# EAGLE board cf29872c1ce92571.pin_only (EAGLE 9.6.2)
REV: E

Size 48.26 x 40.64 mm. Coordinates in mm from the lower left corner, seen from the top.
Outline: 2.54,40.64 45.72,40.64 arc-90 48.26,38.1 48.26,2.54 arc-90 45.72,0 2.54,0 arc-90 0,2.54 0,38.1 arc-90 2.54,40.64
Copper layers (1*16): Top 0.035mm / dielectric 1.5mm / Bottom 0.035mm
Design rules "adafruit 8-8": minimum track width 6mil, minimum drill 15.5mil, track to track 8mil, track to pad 8mil, pad to pad 8mil, via to via 8mil, smd to smd 8mil, copper to edge 10mil, drill to drill 8mil, minimum pad ring 10mil, minimum via ring 8mil, stop-mask expansion 2mil, vias tented up to drill 20mil, thermal gap 10mil

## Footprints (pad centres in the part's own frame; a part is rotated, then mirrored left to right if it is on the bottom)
0603-NO = smd 1.075 x 1: 1 -0.85,0; 2 0.85,0
0805-NO = smd 1.24 x 1.5: 1 -0.95,0; 2 0.95,0
SOD-123 = smd 1.4 x 1.4: A 1.85,0; C -1.85,0
SOD-323_MINI = smd 0.9 x 0.8: A 1.07,0; C -1.07,0
FIDUCIAL_1MM = smd 1 x 1: 1 0,0
SOT23-5 = smd 0.69 x 0.99: 1 -0.95,-1.29; 2 0,-1.29; 3 0.95,-1.29; 4 0.95,1.3; 5 -0.95,1.3
FPC_40 = smd 0.275 x 1.2: 1 -9.75,-1.044; 2 -9.25,-1.044; 3 -8.75,-1.044; 4 -8.25,-1.044; 5 -7.75,-1.044; 6 -7.25,-1.044; 7 -6.75,-1.044; 8 -6.25,-1.044; 9 -5.75,-1.044; 10 -5.25,-1.044; 11 -4.75,-1.044; 12 -4.25,-1.044; 13 -3.75,-1.044; 14 -3.25,-1.044; 15 -2.75,-1.044; 16 -2.25,-1.044; 17 -1.75,-1.044; 18 -1.25,-1.044; 19 -0.75,-1.044; 20 -0.25,-1.044; 21 0.25,-1.044; 22 0.75,-1.044; 23 1.25,-1.044; 24 1.75,-1.044; 25 2.25,-1.044; 26 2.75,-1.044; 27 3.25,-1.044; 28 3.75,-1.044; 29 4.25,-1.044; 30 4.75,-1.044; 31 5.25,-1.044; 32 5.75,-1.044; 33 6.25,-1.044; 34 6.75,-1.044; 35 7.25,-1.044; 36 7.75,-1.044; 37 8.25,-1.044; 38 8.75,-1.044; 39 9.25,-1.044; 40 9.75,-1.044 | smd 2.4 x 3.81: PAD1 11.85,1.163; PAD2 -11.85,1.163
1X15-CB = drill 1.016 pad 1.778: 1 -17.78,0; 2 -15.24,0; 3 -12.7,0; 4 -10.16,0; 5 -7.62,0; 6 -5.08,0; 7 -2.54,0; 8 0,0; 9 2.54,0; 10 5.08,0; 11 7.62,0; 12 10.16,0; 13 12.7,0; 14 15.24,0; 15 17.78,0
INDUCTOR_5X5MM_NR5040_NOTHERMALS = smd 1.8 x 4: P$1 -1.8,0; P$2 1.8,0
RESPACK_4X0603 = smd 0.45 x 0.9: 1 -1.3,-0.85; 2 -0.4,-0.85; 3 0.4,-0.85; 4 1.3,-0.85; 5 1.3,0.85; 6 0.4,0.85; 7 -0.4,0.85; 8 -1.3,0.85
SOLDERJUMPER_ARROW_NOPASTE = smd 0.762 x 1.524: 1 -1.016,0; 2 1.016,0
LQFP100 = smd 0.27 x 1.5: 1 -6,-7.75; 2 -5.5,-7.75; 3 -5,-7.75; 4 -4.5,-7.75; 5 -4,-7.75; 6 -3.5,-7.75; 7 -3,-7.75; 8 -2.5,-7.75; 9 -2,-7.75; 10 -1.5,-7.75; 11 -1,-7.75; 12 -0.5,-7.75; 13 0,-7.75; 14 0.5,-7.75; 15 1,-7.75; 16 1.5,-7.75; 17 2,-7.75; 18 2.5,-7.75; 19 3,-7.75; 20 3.5,-7.75; 21 4,-7.75; 22 4.5,-7.75; 23 5,-7.75; 24 5.5,-7.75; 25 6,-7.75; 51 6,7.75; 52 5.5,7.75; 53 5,7.75; 54 4.5,7.75; 55 4,7.75; 56 3.5,7.75; 57 3,7.75; 58 2.5,7.75; 59 2,7.75; 60 1.5,7.75; 61 1,7.75; 62 0.5,7.75; 63 0,7.75; 64 -0.5,7.75; 65 -1,7.75; 66 -1.5,7.75; 67 -2,7.75; 68 -2.5,7.75; 69 -3,7.75; 70 -3.5,7.75; 71 -4,7.75; 72 -4.5,7.75; 73 -5,7.75; 74 -5.5,7.75; 75 -6,7.75 | smd 1.5 x 0.27: 26 7.75,-6; 27 7.75,-5.5; 28 7.75,-5; 29 7.75,-4.5; 30 7.75,-4; 31 7.75,-3.5; 32 7.75,-3; 33 7.75,-2.5; 34 7.75,-2; 35 7.75,-1.5; 36 7.75,-1; 37 7.75,-0.5; 38 7.75,0; 39 7.75,0.5; 40 7.75,1; 41 7.75,1.5; 42 7.75,2; 43 7.75,2.5; 44 7.75,3; 45 7.75,3.5; 46 7.75,4; 47 7.75,4.5; 48 7.75,5; 49 7.75,5.5; 50 7.75,6; 76 -7.75,6; 77 -7.75,5.5; 78 -7.75,5; 79 -7.75,4.5; 80 -7.75,4; 81 -7.75,3.5; 82 -7.75,3; 83 -7.75,2.5; 84 -7.75,2; 85 -7.75,1.5; 86 -7.75,1; 87 -7.75,0.5; 88 -7.75,0; 89 -7.75,-0.5; 90 -7.75,-1; 91 -7.75,-1.5; 92 -7.75,-2; 93 -7.75,-2.5; 94 -7.75,-3; 95 -7.75,-3.5; 96 -7.75,-4; 97 -7.75,-4.5; 98 -7.75,-5; 99 -7.75,-5.5; 100 -7.75,-6
SC70-5 = smd 0.35 x 1.15: 1 -0.65,-0.85; 2 0,-0.85; 3 0.65,-0.85; 4 0.65,0.85; 5 -0.65,0.85
SOT23-5' = smd 0.55 x 1.2: 1 -0.95,-1.3; 2 0,-1.3; 3 0.95,-1.3; 4 0.95,1.3; 5 -0.95,1.3
TSSOP16 = smd 0.305 x 0.991: 1 -2.275,-2.918; 2 -1.625,-2.918; 3 -0.975,-2.918; 4 -0.325,-2.918; 5 0.325,-2.918; 6 0.975,-2.918; 7 1.625,-2.918; 8 2.275,-2.918; 9 2.275,2.918; 10 1.625,2.918; 11 0.975,2.918; 12 0.325,2.918; 13 -0.325,2.918; 14 -0.975,2.918; 15 -1.625,2.918; 16 -2.275,2.918
MOUNTINGHOLE_2.5_PLATED = drill 2.5 pad 3.2: P$1 0,0
CRYSTAL_3.2X2.5 = smd 1.4 x 1.2: 1 -1.1,-0.8; 2 1.1,0.8; GND1 -1.1,0.8; GND2 1.1,-0.8

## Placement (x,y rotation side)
C1  0.1uF  [0603-NO]  15.24,28.07 90 top
C2  15pF  [0603-NO]  9.9,14.73 0 top
C3  15pF  [0603-NO]  13.58,10.67 180 top
C4  1uF  [0805-NO]  13.96,20.95 180 top
C5  0.1uF  [0603-NO]  36.95,17.4 0 top
C6  0.1uF  [0603-NO]  34.92,9.65 0 top
C7  0.1uF  [0603-NO]  16.25,8.38 180 top
C8  0.1uF  [0603-NO]  37.33,23.24 270 top
C9  0.1uF  [0603-NO]  12.44,8.38 180 top
C10  0.1uF  [0603-NO]  13.96,18.8 180 top
C11  0.1uF  [0603-NO]  13.96,17.27 180 top
C12  0.1uF  [0603-NO]  36.82,15.11 0 top
C16  10uF  [0805-NO]  7.87,17.78 0 top
C17  1uF  [0805-NO]  13.6,24.64 270 top
C18  0.1uF  [0603-NO]  2.41,26.3 0 top
C19  10uF  [0805-NO]  2.28,11.43 90 top
C20  1uF  [0805-NO]  16.76,29.72 270 top
C21  10uF  [0805-NO]  14.16,33.07 180 top
C22  10uF  [0805-NO]  8.63,10.67 90 top
D2  MBR0540  [SOD-123]  11.68,24.51 270 top
D3  1N4148  [SOD-323_MINI]  3.3,17.53 90 top
D4  1N4148  [SOD-323_MINI]  1.52,17.53 90 top
FB2  Ferrite  [0805-NO]  6.35,7.87 270 top
FID1  FIDUCIAL_1MM  [FIDUCIAL_1MM]  2.41,7.11 0 top
FID2  FIDUCIAL_1MM  [FIDUCIAL_1MM]  45.97,7.11 0 top
FID3  FIDUCIAL_1MM  [FIDUCIAL_1MM]  46.35,27.56 0 top
IC2  74AHC1G125DBV  [SOT23-5]  41.02,14.61 270 top
J1  40PINFPC_GENERIC  [FPC_40]  28.44,36.07 0 top
JP1  Breakout  [1X15-CB]  24.13,1.91 180 top
L1  6.8uH large inductor  [INDUCTOR_5X5MM_NR5040_NOTHERMALS]  7.36,21.84 90 top
PLABEL0  [PLABEL0]  6.34,3.05 90 top
PLABEL1  [PLABEL1]  8.88,3.05 90 top
PLABEL2  [PLABEL2]  11.42,2.92 90 top
PLABEL3  [PLABEL3]  16.5,2.92 90 top
PLABEL4  [PLABEL4]  19.04,2.92 90 top
PLABEL5  [PLABEL5]  21.58,3.05 90 top
PLABEL6  [PLABEL6]  24.12,3.05 90 top
PLABEL7  [PLABEL7]  26.66,3.05 90 top
PLABEL8  [PLABEL8]  29.2,3.05 90 top
PLABEL9  [PLABEL9]  31.74,3.05 90 top
PLABEL10  [PLABEL10]  5.46,37.47 0 top
PLABEL11  [PLABEL11]  1.27,34.54 0 top
PLABEL12  [PLABEL12]  1.65,30.99 0 top
PLABEL13  [PLABEL13]  34.28,3.05 90 top
PLABEL14  [PLABEL14]  36.82,3.05 90 top
PLABEL15  [PLABEL15]  39.36,3.05 90 top
PLABEL16  [PLABEL16]  41.9,3.05 90 top
PLABEL17  [PLABEL17]  13.96,3.05 90 top
PLABEL18  [PLABEL18]  5.33,26.42 0 top
PLABEL19  [PLABEL19]  2.29,32.89 0 top
PLABEL20  [PLABEL20]  9.02,26.42 0 top
PLABEL21  [PLABEL21]  30.1,34.67 0 bottom
PLABEL22  [PLABEL22]  24.77,24.13 0 bottom
PLABEL23  [PLABEL23]  25.02,13.34 0 bottom
R1  2Ω  [0805-NO]  10.67,29.08 90 top
R3  1M  [0603-NO]  10.66,11.68 90 top
R4  33  [RESPACK_4X0603]  32.5,29.21 0 top
R5  33  [RESPACK_4X0603]  28.44,29.21 0 top
R6  33  [RESPACK_4X0603]  24.38,29.21 0 top
R7  33  [RESPACK_4X0603]  20.31,29.46 0 top
R8  33  [RESPACK_4X0603]  36.57,29.21 0 top
R9  8.2Ω  [0805-NO]  6.73,28.96 90 top
R10  8.2Ω  [0805-NO]  2.67,28.96 90 top
R11  10K  [0603-NO]  2.4,20.57 0 top
R12  10K  [0603-NO]  38.98,10.41 90 top
SJ1  +25mA  [SOLDERJUMPER_ARROW_NOPASTE]  4.7,28.96 90 top
SJ2  +100mA  [SOLDERJUMPER_ARROW_NOPASTE]  8.76,28.96 90 top
U1  RA8875  [LQFP100]  25.65,17.02 0 top
U3  TPS61169  [SC70-5]  2.28,23.75 180 top
U4  AP2127K-3.3  [SOT23-5']  5.33,11.68 90 top
U5  74HC4050  [TSSOP16]  43.05,19.68 270 top
U$18  [ADAFRUIT_5MM]  43.02,30.76 0 top
U$21  MOUNTINGHOLE2.5  [MOUNTINGHOLE_2.5_PLATED]  2.54,38.1 0 top
U$22  MOUNTINGHOLE2.5  [MOUNTINGHOLE_2.5_PLATED]  45.72,38.1 0 top
U$23  MOUNTINGHOLE2.5  [MOUNTINGHOLE_2.5_PLATED]  45.72,2.54 0 top
U$24  MOUNTINGHOLE2.5  [MOUNTINGHOLE_2.5_PLATED]  2.54,2.54 0 top
U$25  [ADAFRUIT_TEXT_20MM]  35.94,4.32 0 bottom
U$30  [PCBFEAT-REV-040]  13.72,36.2 0 top
Y1  20MHz  [CRYSTAL_3.2X2.5]  13.45,13.72 90 top

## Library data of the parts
C1-C12 C16-C22 D2-D4 FB2 L1 R1 R3-R12 U1 U5 U$18 U$25 U$30 Y1 = microbuilder
FID1-FID3 SJ1 SJ2 = microbuilder; BOM: EXCLUDE
IC2 = 74xx-little-us; ROT: 0
J1 = adafruit_display
JP1 = adafruit
PLABEL0 PLABEL1-PLABEL23 = pinguin
U3 = adafruit_power; ROT: 270
U4 = adafruit_power; JLC_ROTATION: 270
U$21-U$24 = adafruit_electromech; BOM: EXCLUDE

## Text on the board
Pinguin_tBackup: RA8875 | SPI->40p TFT | with Touch | 800x480 max | +25 | +100 | VIN | GND | 3Vo | LITE | SCK | MISO | MOSI | CS | RST | WAIT | INT | Y+ | Y- | X- | X+
Pinguin_bBackup: RA8875 | RGB TFT Driver with SPI Interface / Hardware GFX Accel & Touchscreen / Vin: 3.3-5V in / Logic Level: 3.3-5V / / Backlight: 25mA nominal, 24V peak / Close +25mA/+100 jumpers for C.C. | Max resolution: 800x480 @ 16bpp

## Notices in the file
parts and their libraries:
microbuilder: This work is placed in the public domain, and may be freely used for commercial and non-commercial work with the following conditions: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
